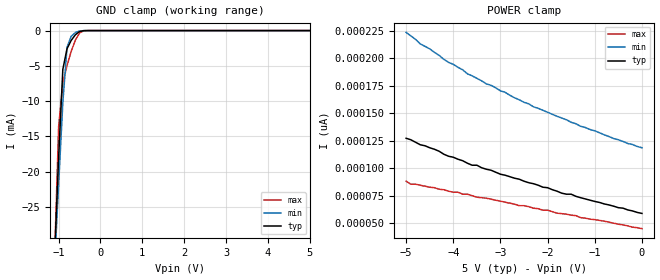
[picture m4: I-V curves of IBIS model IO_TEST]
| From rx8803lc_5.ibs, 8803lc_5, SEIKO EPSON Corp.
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[Model]   IO_TEST
Model_type Input
Enable Active-High
Polarity Non-Inverting
Vinh=4.0
Vinl=1.0
C_comp   5p   4p   6p
[Temperature Range] 25   85   -40
[Voltage Range]   5.0   4.5   5.5
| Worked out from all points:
|   GND clamp passes 1 mA (typ) near -0.65 V on its own axis
[GND Clamp]
-5V       -640.1mA   -524.9mA   -814.3mA
-1.1V     -32.43mA   -33.46mA   -32.61mA
-1V       -17.96mA   -21.79mA   -13.59mA
-900mV    -5.499mA   -10.22mA   -7.421mA
-800mV    -2.576mA   -2.362mA   -4.965mA
-700mV    -1.392mA   -807.3uA   -2.943mA
-600mV    -591.5uA   -281.9uA   -1.347mA
-500mV    -144.6uA   -61.93uA   -343.6uA
-400mV    -15.25uA   -7.313uA   -28.72uA
-300mV    -812.1nA   -557.3nA   -822.7nA
5V        58.89pA    126pA      40.93pA
[POWER Clamp]
-5V       127.3pA    223.7pA    88.22pA
-4.9V     126pA      220.6pA    85.49pA
-4.7V     121.4pA    213.3pA    84.58pA
-4.4V     117.3pA    205.5pA    82.31pA
-4.2V     112.8pA    199.2pA    80.49pA
-3.8V     106.9pA    189.6pA    76.4pA
-3.7V     104.6pA    186pA      76.4pA
-2.7V     90.95pA    164.2pA    67.3pA
-1.7V     77.31pA    145.7pA    58.66pA
-1.5V     76.4pA     141.9pA    57.3pA
-1.3V     73.21pA    138.2pA    55.02pA
0V        58.89pA    118.7pA    45.02pA
